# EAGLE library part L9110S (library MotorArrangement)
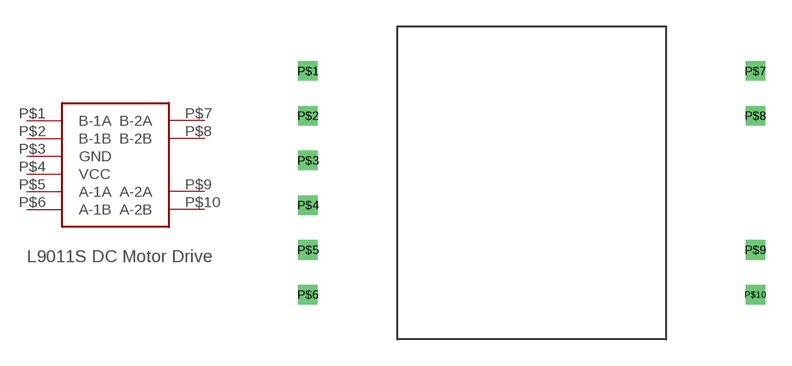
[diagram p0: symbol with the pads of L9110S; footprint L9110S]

Designator prefix -

## L9110S  [L9110S]
P$1  B-1A
P$2  B-1B
P$3  GND
P$4  VCC
P$5  A-1A
P$6  A-1B
P$7  B-2A
P$8  B-2B
P$9  A-2A
P$10  A-2B

## Footprint L9110S (pad centres in mm)
drill 0.6 square: P$1 -12.7,5.08; P$2 -12.7,2.54; P$3 -12.7,0; P$4 -12.7,-2.54; P$5 -12.7,-5.08; P$6 -12.7,-7.62; P$7 12.7,5.08; P$8 12.7,2.54; P$9 12.7,-5.08; P$10 12.7,-7.62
